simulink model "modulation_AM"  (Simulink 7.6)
settings: Solver=ode15s  StartTime=0.0  StopTime=10.0  RelTol=1e-3
libraries: fl_lib x13, nesl_utility x4

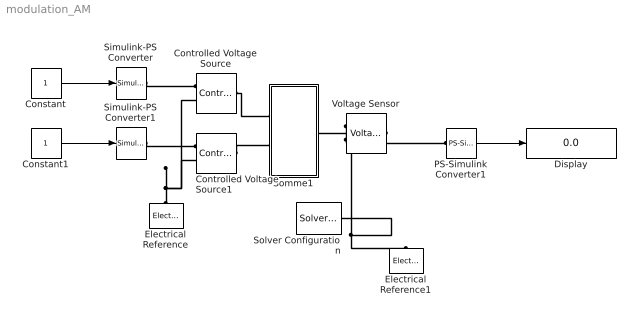
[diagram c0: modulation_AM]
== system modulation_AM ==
  Constant : Constant
  Constant1 : Constant
  Controlled Voltage Source : fl_lib/Electrical/Electrical Sources/Controlled Voltage Source  DialogController=NetworkEngine.DynNeDlgSource  SystemSampleTime=-1  i_Log=off  v_Log=off  LocalVarNames=|i|v  LocalVarDescs=|i|v  LocalVarLogging=[0 0]
  Controlled Voltage Source1 : fl_lib/Electrical/Electrical Sources/Controlled Voltage Source  DialogController=NetworkEngine.DynNeDlgSource  SystemSampleTime=-1  i_Log=off  v_Log=off  LocalVarNames=|i|v  LocalVarDescs=|i|v  LocalVarLogging=[0 0]
  Display : Display
  Electrical Reference : fl_lib/Electrical/Electrical Elements/Electrical Reference  DialogController=NetworkEngine.DynNeDlgSource  SystemSampleTime=-1  i_Log=off  LocalVarNames=|i  LocalVarDescs=|i  LocalVarLogging=0
  Electrical Reference1 : fl_lib/Electrical/Electrical Elements/Electrical Reference  DialogController=NetworkEngine.DynNeDlgSource  SystemSampleTime=-1  i_Log=off  LocalVarNames=|i  LocalVarDescs=|i  LocalVarLogging=0
  PS-Simulink Converter1 : nesl_utility/PS-Simulink Converter  DialogController=NetworkEngine.DynNeUtilDlgSource  SystemSampleTime=-1  PhysicalDomain=network_engine_domain  LeftPortType=input  RightPortType=output  SubClassName=ps_output  Unit=1  AffineConversion=off
  Simulink-PS Converter : nesl_utility/Simulink-PS Converter  DialogController=NetworkEngine.DynNeUtilDlgSource  SystemSampleTime=-1  PhysicalDomain=network_engine_domain  LeftPortType=input  RightPortType=output  SubClassName=ps_input  Unit=1  AffineConversion=off  InputFilterTimeConstant=.001  UdotUserProvided=0
  Simulink-PS Converter1 : nesl_utility/Simulink-PS Converter  DialogController=NetworkEngine.DynNeUtilDlgSource  SystemSampleTime=-1  PhysicalDomain=network_engine_domain  LeftPortType=input  RightPortType=output  SubClassName=ps_input  Unit=1  AffineConversion=off  InputFilterTimeConstant=.001  UdotUserProvided=0
  Solver Configuration : nesl_utility/Solver Configuration  DialogController=NetworkEngine.DynNeUtilDlgSource  SystemSampleTime=-1  PhysicalDomain=network_engine_domain  LeftPortType=input  RightPortType=generic  SubClassName=solver  Accelerate=off  Profile=off  ResidualTolerance=1e-9  MaxNonlinIter=3  MaxModeIter=2  DoFixedCost=off  UseLocalSampling=off  DoDC=off  LinearAlgebra=Sparse  LocalSolverSampleTime=.001  LocalSolverChoice=NE_BACKWARD_EULER_ADVANCER  UseLocalSolver=off
  Somme1 : Subsystem
  Voltage Sensor : fl_lib/Electrical/Electrical Sensors/Voltage Sensor  DialogController=NetworkEngine.DynNeDlgSource  SystemSampleTime=-1  i1_Log=off  v1_Log=off  LocalVarNames=|i1|v1  LocalVarDescs=|i1|v1  LocalVarLogging=[0 0]
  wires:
  Constant/1 -> Simulink-PS Converter/1
  Constant1/1 -> Simulink-PS Converter1/1
  PS-Simulink Converter1/1 -> Display/1
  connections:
  Controlled Voltage Source/LConn1 -- Somme1/LConn1
  Simulink-PS Converter/RConn1 -- Controlled Voltage Source/RConn1
  Simulink-PS Converter1/RConn1 -- Controlled Voltage Source1/RConn1
  Controlled Voltage Source1/LConn1 -- Somme1/LConn2
  Electrical Reference/LConn1 -- Controlled Voltage Source1/RConn2 -- Controlled Voltage Source/RConn2
  Somme1/RConn1 -- Voltage Sensor/LConn1
  Voltage Sensor/RConn1 -- PS-Simulink Converter1/LConn1
  Voltage Sensor/RConn2 -- Electrical Reference1/LConn1 -- Solver Configuration/RConn1

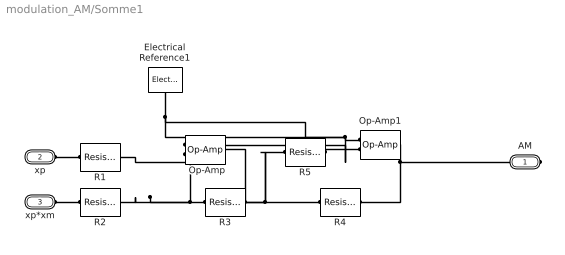
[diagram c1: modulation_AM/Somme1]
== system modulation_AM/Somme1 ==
  Electrical Reference1 : fl_lib/Electrical/Electrical Elements/Electrical Reference  DialogController=NetworkEngine.DynNeDlgSource  SystemSampleTime=-1  i_Log=off  LocalVarNames=|i  LocalVarDescs=|i  LocalVarLogging=0
  Op-Amp : fl_lib/Electrical/Electrical Elements/Op-Amp  DialogController=NetworkEngine.DynNeDlgSource  SystemSampleTime=-1  i1_Log=off  v1_Log=off  outI_Log=off  LocalVarNames=|i1|v1|outI  LocalVarDescs=|i1|v1|outI  LocalVarLogging=[0 0 0]
  Op-Amp1 : fl_lib/Electrical/Electrical Elements/Op-Amp  DialogController=NetworkEngine.DynNeDlgSource  SystemSampleTime=-1  i1_Log=off  v1_Log=off  outI_Log=off  LocalVarNames=|i1|v1|outI  LocalVarDescs=|i1|v1|outI  LocalVarLogging=[0 0 0]
  R1 : fl_lib/Electrical/Electrical Elements/Resistor  DialogController=NetworkEngine.DynNeDlgSource  SystemSampleTime=-1  R=1 Ohm  i_Log=off  v_Log=off  LocalVarNames=|i|v  LocalVarDescs=|i|v  LocalVarLogging=[0 0]
  R2 : fl_lib/Electrical/Electrical Elements/Resistor  DialogController=NetworkEngine.DynNeDlgSource  SystemSampleTime=-1  R=1 Ohm  i_Log=off  v_Log=off  LocalVarNames=|i|v  LocalVarDescs=|i|v  LocalVarLogging=[0 0]
  R3 : fl_lib/Electrical/Electrical Elements/Resistor  DialogController=NetworkEngine.DynNeDlgSource  SystemSampleTime=-1  R=1 Ohm  i_Log=off  v_Log=off  LocalVarNames=|i|v  LocalVarDescs=|i|v  LocalVarLogging=[0 0]
  R4 : fl_lib/Electrical/Electrical Elements/Resistor  DialogController=NetworkEngine.DynNeDlgSource  SystemSampleTime=-1  R=1 kOhm  i_Log=off  v_Log=off  LocalVarNames=|i|v  LocalVarDescs=|i|v  LocalVarLogging=[0 0]
  R5 : fl_lib/Electrical/Electrical Elements/Resistor  DialogController=NetworkEngine.DynNeDlgSource  SystemSampleTime=-1  R=1 kOhm  i_Log=off  v_Log=off  LocalVarNames=|i|v  LocalVarDescs=|i|v  LocalVarLogging=[0 0]
  AM : PMIOPort  Port=1  Side=Right
  xp : PMIOPort  Port=2  Side=Left
  xp*xm : PMIOPort  Port=3  Side=Left
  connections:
  R5/RConn1 -- Op-Amp1/LConn2
  R4/RConn1 -- AM/RConn1 -- Op-Amp1/RConn1
  xp*xm/RConn1 -- R2/LConn1
  xp/RConn1 -- R1/LConn1
  R3/RConn1 -- R5/LConn1 -- Op-Amp/RConn1 -- R4/LConn1
  R3/LConn1 -- Op-Amp/LConn2 -- R1/RConn1 -- R2/RConn1
  Op-Amp1/LConn1 -- Op-Amp/LConn1 -- Electrical Reference1/LConn1
